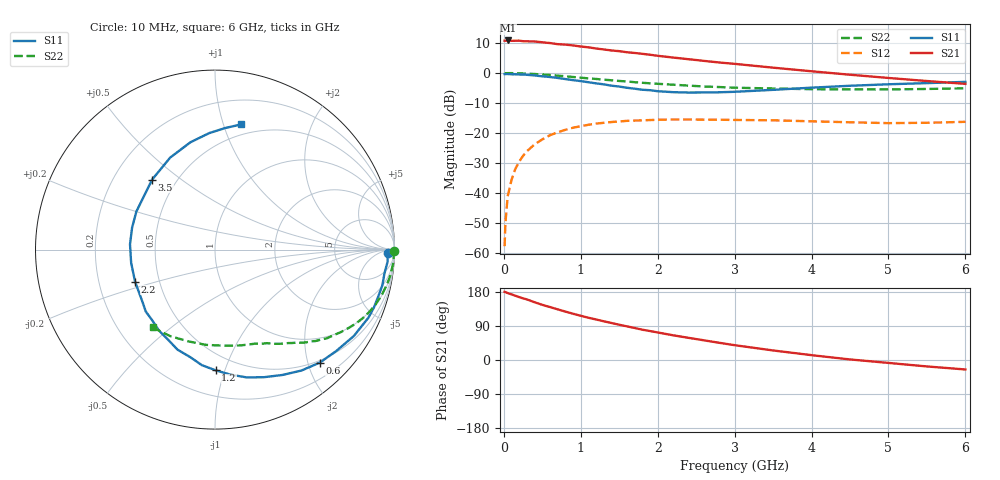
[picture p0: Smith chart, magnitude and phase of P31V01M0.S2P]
! SIEMENS Small Signal Semiconductors
! BFP181
! Si NPN RF Bipolar Junction Transistor in SOT143
! VCE = 1 V  IC = 1 mA
! Common Emitter S-Parameters:  March  1996
# GHz  S  MA  R  50
!  f  S11  S21  S12  S22
! GHz  MAG  ANG  MAG  ANG  MAG  ANG  MAG  ANG
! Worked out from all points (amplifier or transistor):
!   36 points, 10 MHz to 6 GHz, reference 50 ohm
!   highest |S21| = 10.9 dB at 50 MHz (marker M1)
!   |S21| within 3 dB of that: start of sweep to 1.299 GHz
!   unconditionally stable (mu >= 1): 2.915 GHz to end of sweep
!   at 250 MHz: K = 0.10, MSG = 19.1 dB, |S12| = -27.6 dB
!   at 1.4 GHz: K = 0.53, MSG = 11.9 dB, |S12| = -16.3 dB
!   at 6 GHz: K = 1.36, MAG = 2.8 dB, |S12| = -16.3 dB
!   S11 on the Smith chart (normalised r, x): 10 MHz: 43, -19; 600 MHz: 0.46, -2.21; 1.2 GHz: 0.38, -0.93; 2.2 GHz: 0.36, -0.17; 3.5 GHz: 0.37, +0.40; 6 GHz: 0.40, +1.15
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0.01  0.9616 -1.0  3.462 179.7  0.0013 85.4  0.9977 -0.3
0.02  0.9622 -1.6  3.447 179.3  0.0031 85.4  0.9937 -0.8
0.05  0.9641 -4.0  3.492 176.6  0.0088 89.0  0.9955 -2.0
0.1  0.9532 -8.1  3.443 173.1  0.0166 84.1  0.9965 -3.9
0.15  0.9535 -12.0  3.45 169.6  0.0253 81.8  0.9921 -5.8
0.2  0.9461 -16.3  3.466 166.0  0.0335 78.9  0.9888 -7.8
0.25  0.9425 -19.9  3.394 162.6  0.0417 76.8  0.9829 -9.8
0.4  0.9112 -31.9  3.359 152.3  0.0646 69.1  0.9632 -15.2
0.5  0.8807 -39.9  3.255 145.5  0.0783 63.8  0.946 -18.8
0.6  0.8589 -47.1  3.16 139.7  0.0919 59.1  0.9266 -22.1
0.8  0.7932 -61.7  2.976 127.7  0.113 50.6  0.8837 -28.0
0.9  0.7615 -69.0  2.883 122.0  0.1227 46.4  0.8597 -30.8
1.1  0.7021 -82.9  2.682 111.5  0.1374 39.2  0.8152 -35.8
1.2  0.6726 -89.7  2.563 106.9  0.1436 35.4  0.7965 -38.3
1.5  0.5954 -110.5  2.315 93.0  0.1558 27.3  0.7375 -43.9
1.8  0.5266 -131.7  2.089 80.0  0.1629 20.5  0.6882 -48.9
2.2  0.4798 -158.2  1.813 65.2  0.1681 12.5  0.6389 -55.2
2.8  0.4778 165.2  1.499 45.4  0.1666 4.3  0.5843 -63.9
3.5  0.5244 131.9  1.229 25.2  0.163 -2.3  0.5526 -75.1
4.5  0.6134 102.9  0.937 1.5  0.1511 -7.1  0.5331 -95.4
5.5  0.6792 85.3  0.736 -17.0  0.1482 -4.9  0.5428 -117.4
6  0.7126 78.2  0.66 -25.0  0.1537 -4.0  0.5558 -128.7
